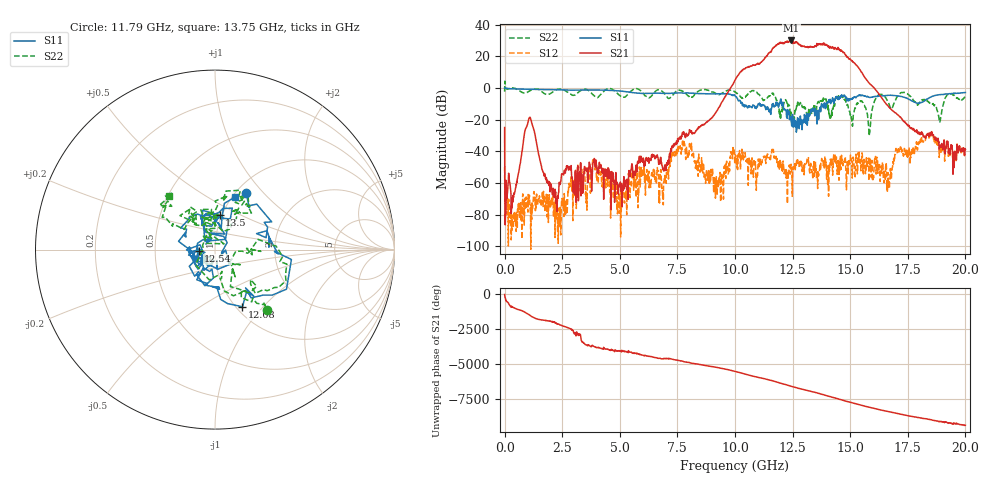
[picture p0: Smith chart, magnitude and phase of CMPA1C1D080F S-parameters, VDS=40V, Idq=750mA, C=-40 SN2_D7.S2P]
!Keysight Technologies,E5071C,MY46632380,B.14.03
!Date: Tue Nov 10 04:55:51 2020
!Data & Calibration Information:
!Freq	S11:SOLT2(ON)	S21:SOLT2(ON)	S12:SOLT2(ON)	S22:SOLT2(ON)
!PortZ  Port1:50+j0  Port2:50+j0
!Above PortZ is port z conversion or system Z0 setting when saving the data.
!When reading, reference impedance value at option line is always used.
# Hz S dB R 50
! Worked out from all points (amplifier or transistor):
!   1601 points, 300 kHz to 20 GHz, reference 50 ohm
!   highest |S21| = 30.1 dB at 12.45 GHz (marker M1)
!   |S21| within 3 dB of that: 11.81 GHz to 12.84 GHz (1.031 GHz wide, 8.37 % of centre)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
!   unconditionally stable (mu >= 1): 49.13 MHz to 276.9 MHz; 371.4 MHz to 381.6 MHz; 392.1 MHz to end of sweep
!   at 3.325 GHz: K = 9652.66, MAG = -43.9 dB, |S12| = -53.4 dB
!   at 10 GHz: K = 13.26, MAG = 10.5 dB, |S12| = -44.5 dB
!   at 20 GHz: K = 1208.37, MAG = -33.8 dB, |S12| = -38.7 dB
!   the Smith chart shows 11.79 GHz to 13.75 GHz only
!   S11 on the Smith chart (normalised r, x): 11.79 GHz: 1.11, +0.80; 12.08 GHz: 1.07, -0.78; 12.54 GHz: 0.83, -0.01; 13.5 GHz: 0.98, +0.39; 13.75 GHz: 1.03, +0.67
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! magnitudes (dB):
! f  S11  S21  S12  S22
! 300 kHz  0.0  -25.0  -49.8  -2.3
! 112.8 MHz  -0.2  -67.9  -70.3  -0.7
! 387.8 MHz  -0.6  -69.1  -85.0  0.0
! 1.1 GHz  -0.8  -18.5  -74.5  -1.7
! 2.213 GHz  -1.1  -65.6  -70.6  -1.3
! 2.675 GHz  -1.2  -51.0  -72.0  -2.1
! 3.338 GHz  -1.3  -54.4  -51.6  -1.3
! 4.963 GHz  -1.8  -61.4  -66.1  -4.3
! 6.675 GHz  -3.3  -46.2  -54.7  -1.1
! 7.713 GHz  -3.1  -28.5  -34.7  -1.9
! 9.3 GHz  -3.6  -12.3  -59.7  -4.1
! 10 GHz  -4.8  4.9  -44.5  -2.4
! 11.79 GHz  -8.9  27.3  -43.2  -7.1
! 12.08 GHz  -9.0  28.3  -48.2  -14.0
! 12.45 GHz  -22.1  30.1  -51.5  -17.3
! 12.54 GHz  -20.8  28.7  -51.3  -24.4
! 13.34 GHz  -14.6  26.1  -53.4  -16.4
! 13.5 GHz  -14.3  26.4  -49.2  -13.2
! 13.75 GHz  -10.1  27.4  -46.7  -8.1
! 16.68 GHz  -4.6  -11.9  -62.3  -9.7
! 18.39 GHz  -6.6  -28.7  -29.7  -8.8
! 20 GHz  -2.8  -38.7  -38.7  -5.1
